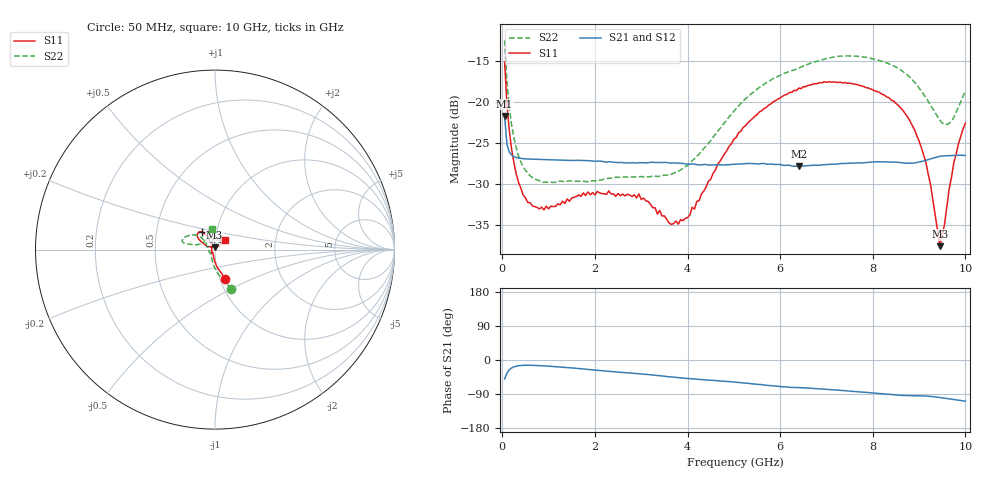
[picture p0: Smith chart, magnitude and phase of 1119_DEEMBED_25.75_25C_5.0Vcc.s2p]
!Hittite Microwave Corp.
!Digital Attenuator/PhaseShifter Rev 1.4.0
!Filename: C:\DATA\DATA\1119_DEEMBED_25.75_25C_5.0Vcc.s2p
!VNA ID: Agilent Technologies,N5224A,MY51441122,A.10.45.03
!Device type:
!2 Port Calibration.
!Temp(C): 25
!Lot Number:
!Serial Number:
!Operator:
!Misc:
!Attenuator:  25.750
# GHZ S DB R 50.0
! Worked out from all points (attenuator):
!   200 points, 50 MHz to 10 GHz, reference 50 ohm
!   highest |S21| = -21.74 dB at 50 MHz (marker M1); lowest = -27.8 dB at 6.4 GHz (marker M2)
!   lowest |S11| = -37.5 dB at 9.45 GHz (marker M3), VSWR 1.03, Z = 49.7 + j1.29 ohm
!   |S11| at or under -10 dB: start of sweep to end of sweep
!   |S22| runs from -29.8 to -12.6 dB; largest |S21 - S12| = 0.00015
!   S11 on the Smith chart (normalised r, x): 50 MHz: 1.06, -0.36; 6.4 GHz: 0.85, +0.17; 10 GHz: 1.11, +0.11
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0.05  -15.17 -70.4  -21.74 -50.1  -21.73 -50.1  -12.56 -67.3
0.1  -20.30 -83.5  -25.14 -34.6  -25.14 -34.7  -17.51 -83.9
0.2  -25.70 -95.8  -26.47 -21.0  -26.47 -21.0  -22.79 -100.5
0.45  -31.30 -111.7  -26.91 -14.1  -26.90 -14.1  -27.87 -121.2
0.9  -33.13 -126.0  -27.03 -15.5  -27.03 -15.5  -29.77 -135.7
1.75  -31.07 -133.4  -27.13 -23.8  -27.13 -23.8  -29.65 -140.7
2.95  -31.19 -134.1  -27.39 -36.2  -27.39 -36.2  -29.10 -159.9
3.4  -33.19 -153.5  -27.38 -41.4  -27.38 -41.5  -29.03 -173.4
3.65  -34.89 -173.5  -27.45 -44.5  -27.46 -44.6  -28.79 177.4
4  -34.07 151.4  -27.57 -48.8  -27.58 -48.8  -27.75 162.2
5.05  -24.34 118.0  -27.57 -58.5  -27.60 -58.6  -20.83 138.8
5.55  -21.24 119.8  -27.55 -64.5  -27.56 -64.6  -18.26 141.2
6.4  -18.34 126.0  -27.84 -72.8  -27.86 -72.9  -15.92 150.0
6.7  -17.88 129.7  -27.71 -74.9  -27.72 -74.9  -15.24 153.9
7.5  -17.73 139.9  -27.47 -82.2  -27.47 -82.2  -14.44 163.6
8.35  -19.51 147.3  -27.32 -90.8  -27.32 -90.8  -15.39 168.1
8.75  -21.83 151.4  -27.46 -93.8  -27.46 -93.8  -16.76 168.1
9.05  -25.57 155.0  -27.25 -94.5  -27.25 -94.5  -18.71 166.9
9.25  -30.14 151.8  -26.93 -96.1  -26.94 -96.1  -20.44 162.2
9.45  -37.53 101.7  -26.62 -99.1  -26.63 -99.1  -22.24 149.3
9.75  -27.38 40.9  -26.52 -104.2  -26.52 -104.2  -21.88 114.3
10  -22.61 43.8  -26.53 -108.6  -26.53 -108.6  -18.65 98.5
